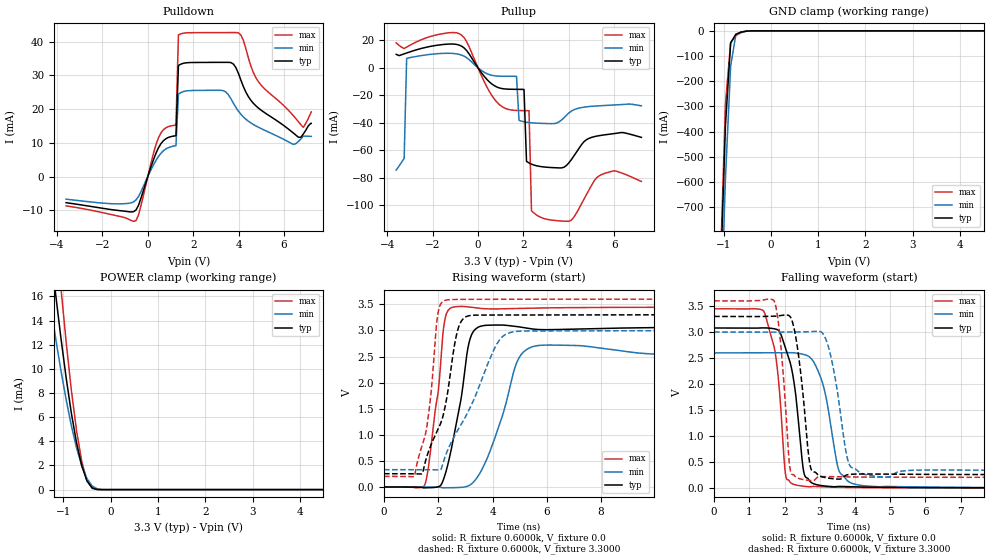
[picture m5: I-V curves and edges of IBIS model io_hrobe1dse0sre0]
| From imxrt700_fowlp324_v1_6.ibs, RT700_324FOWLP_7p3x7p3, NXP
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[Model] io_hrobe1dse0sre0
|   Model io_hrobe1dse0sre0
| This model was characterised for following simulation conditions:
| External (pad) voltage:
|   - Typ: 3.3V,   - Min: 3.0V,   - Max: 3.6V
| Library cells for typ/min/max conditions are connected as defined below:
|  PAD_IO - External Pad
|  ipp_do - Core Input
|  ipp_obe - Output Buffer Enable
|  ASRCN3V3[3] - NC
|  ASRCN3V3[4] - NC
|  ASRCP3V3[4] - NC
|  REFAPBIAS3V3 - gnde
|  REFBAMPL3V3 - vdd1v8
|  REFCAMPH3V3 - vdd1v8
|  REFDNBIAS3V3 - vdd1v8
|  REFH3V3 - REFH3V3
|  REFL3V3 - REFL3V3
|  gnde - gnde
|  ipp_dse - gnde
|  ipp_ina235_3v - NC
|  ipp_ina40_3v - NC
|  ipp_ina_mux - NC
|  ipp_ind - NC
|  ipp_ind_1p8v - NC
|  ipp_ind_3v - NC
|  ipp_sre - gnde
|  vdd - vdd
|  vdd1v8 - vdd1v8
|  vdda - vdde3v3
|  vdde3v3 - vdde3v3
| All other pins connected to ground
Model_type I/O
Polarity   Non-Inverting
Enable   Active-High
Vinl =   0.9900V
Vinh =   2.3100V
Vmeas =  1.6500V
Cref =   15.0000pF
Rref =   0.6000k
Vref =   0.0V
C_comp   4.0008pF   3.8189pF   4.1206pF
|C_comp_pullup   0.5645pF   0.7341pF   0.4703pF
|C_comp_pulldown   2.1156pF   2.2138pF   1.8992pF
[Model Spec]
| variable   typ   min   max
Vinh   2.3100V   NA   NA
Vinl   0.9900V   NA   NA
Vref   0.0V   0.0V   0.0V
Cref   15.0000pF   15.0000pF   15.0000pF
Rref   0.6000k   0.6000k   0.6000k
[Receiver Thresholds]
Vcross_high  =   0.0V
Vcross_low  =   0.0V
Vdiff_ac  =   0.0V
Vdiff_dc  =   0.0V
Tdiffslew_ac  =   0.0S
[Temperature Range]   25.0000   0.1250k   -40.0000
[Voltage Range]   3.3000V   3.0000V   3.6000V
[Pullup Reference]   3.3000V   3.0000V   3.6000V
[Pulldown Reference]   0.0V   0.0V   0.0V
[POWER Clamp Reference]   3.3000V   3.0000V   3.6000V
[GND Clamp Reference]   0.0V   0.0V   0.0V
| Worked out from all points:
|   slope of the pulldown table from 0 to 0.495 V, typ, clamps not added: 56.2 ohm
|   slope of the pullup table from 0 to 0.495 V, typ, clamps not added: 48.6 ohm
|   GND clamp passes 1 mA (typ) near -0.49 V on its own axis
|   POWER clamp passes 1 mA (typ) near -0.52 V on its own axis
|   rising waveform, R_fixture 0.6000k, V_fixture 0.0: 20-80 % time 596ps typ, 935ps min, 426ps max; typ from 0 V to 3.08 V
|   rising waveform, R_fixture 0.6000k, V_fixture 3.3000: 20-80 % time 811ps typ, 1.42ns min, 442ps max; typ from 0.254 V to 3.3 V
|   falling waveform, R_fixture 0.6000k, V_fixture 0.0: 20-80 % time 347ps typ, 425ps min, 283ps max; typ from 3.08 V to 0 V
|   falling waveform, R_fixture 0.6000k, V_fixture 3.3000: 20-80 % time 278ps typ, 365ps min, 222ps max; typ from 3.3 V to 0.254 V
[Pulldown]
|Voltage   I(typ)   I(min)   I(max)
-3.6V     -7.76mA    -6.72mA    -8.7mA
-520mV    -9.932mA   -6.949mA   -13.06mA
470mV     8.52mA     5.95mA     11.5mA
1.24V     12.09mA    9.145mA    15.23mA
1.35V     32.94mA    24.47mA    42.02mA
1.46V     33.35mA    24.92mA    42.34mA
3.33V     33.87mA    25.46mA    42.7mA
3.99V     30.63mA    19.41mA    42.61mA
5.09V     19.21mA    13.9mA     26.38mA
6.41V     12.92mA    9.507mA    18.07mA
6.85V     12.6mA     11.99mA    14.58mA
7.2V      15.78mA    11.9mA     19.19mA
[Pullup]
|Voltage   I(typ)   I(min)   I(max)
-3.6V     9.752mA    -74.51mA   18.1mA
-3.25V    10.1mA     -65.93mA   14.02mA
-3.14V    10.73mA    6.826mA    15.05mA
-830mV    16.51mA    9.731mA    24.85mA
1.7V      -15.72mA   -6.278mA   -31.08mA
1.81V     -15.74mA   -38.27mA   -31.14mA
2.03V     -15.78mA   -39.34mA   -31.22mA
2.14V     -68.17mA   -39.67mA   -31.25mA
2.25V     -69.31mA   -39.91mA   -31.27mA
2.36V     -70.19mA   -40.09mA   -104.1mA
2.69V     -71.74mA   -40.43mA   -108.3mA
7.2V      -50.7mA    -27.72mA   -82.8mA
[GND_clamp]
|Voltage   I(typ)   I(min)   I(max)
-3.6V     -19.67A    -19.55A    -20.65A
-1.07V    -1.013A    -1.224A    -956.3mA
-960mV    -377.1mA   -587.4mA   -291.7mA
-850mV    -48.21mA   -140.8mA   -46.94mA
-740mV    -13.57mA   -15.59mA   -19.22mA
-630mV    -5.137mA   -4.351mA   -7.235mA
-520mV    -1.276mA   -1.53mA    -1.554mA
-300mV    -4.403uA   -32.47uA   -997nA
7.2V      0A         0A         0A
[POWER_clamp]
|Voltage   I(typ)   I(min)   I(max)
-3.6V     102.5mA    81.21mA    131.1mA
-1.38V    23.81mA    18.18mA    31.78mA
-1.27V    19.88mA    15.26mA    26.56mA
-1.16V    16.12mA    12.48mA    21.52mA
-1.05V    12.56mA    9.868mA    16.71mA
-830mV    6.344mA    5.304mA    8.253mA
-720mV    3.878mA    3.458mA    4.888mA
-610mV    1.973mA    1.979mA    2.327mA
-500mV    725uA      918.2uA    733.4uA
-390mV    144.3uA    301.5uA    95.95uA
-170mV    198.2nA    4.056uA    20.28nA
7.2V      0A         0A         0A
[Ramp]
| variable   typ   min   max
dV/dt_r  1.8464/0.5956n   1.5590/0.9347n   2.0681/0.4255n
dV/dt_f  1.8274/0.2775n   1.6009/0.3654n   2.0384/0.2219n
R_load = 0.6000k
[Rising Waveform]
R_fixture= 0.6000k
V_fixture= 0.0
V_fixture_min= 0.0
V_fixture_max= 0.0
|time   V(typ)   V(min)   V(max)
0s        180nV      2.945uV    139nV
1.511ns   -16.45mV   -832.6uV   46.91mV
1.996ns   3.716mV    -4.935mV   1.812V
2.224ns   187.6mV    -16.17mV   3.147V
2.657ns   1.198V     -12.73mV   3.456V
3.104ns   2.689V     19.88mV    3.451V
3.341ns   3.009V     117.6mV    3.438V
4.935ns   3.072V     2.432V     3.422V
5.73ns    3.017V     2.713V     3.43V
60ns      3.077V     2.598V     3.447V
[Rising Waveform]
R_fixture= 0.6000k
V_fixture= 3.3000
V_fixture_min= 3.0000
V_fixture_max= 3.6000
|time   V(typ)   V(min)   V(max)
0s        254.3mV    331.8mV    202.7mV
1.129ns   253.9mV    331.7mV    211.9mV
1.608ns   628.1mV    331.7mV    1.251V
1.994ns   1.108V     327.7mV    3.338V
2.384ns   1.94V      751mV      3.589V
2.675ns   2.918V     1.047V     3.594V
2.917ns   3.223V     1.261V     3.595V
4.139ns   3.295V     2.721V     3.596V
4.896ns   3.295V     2.982V     3.598V
60ns      3.3V       3V         3.6V
[Falling Waveform]
R_fixture= 0.6000k
V_fixture= 0.0
V_fixture_min= 0.0
V_fixture_max= 0.0
|time   V(typ)   V(min)   V(max)
0s        3.077V     2.599V     3.447V
1.406ns   3.08V      2.599V     3.403V
1.861ns   3.003V     2.598V     1.829V
2.049ns   2.647V     2.603V     191.1mV
2.534ns   350.7mV    2.571V     31.8mV
2.672ns   173.3mV    2.536V     21.7mV
3.123ns   37.11mV    1.911V     18.6mV
3.557ns   27.27mV    311.7mV    10.01mV
4.49ns    12.42mV    28.03mV    3.324mV
60ns      676.4nV    2.172uV    497.9nV
[Falling Waveform]
R_fixture= 0.6000k
V_fixture= 3.3000
V_fixture_min= 3.0000
V_fixture_max= 3.6000
|time   V(typ)   V(min)   V(max)
0s        3.3V       3V         3.6V
1.715ns   3.303V     3V         3.583V
1.886ns   3.317V     2.998V     2.804V
2.164ns   3.292V     3.001V     335.7mV
2.388ns   2.6V       3.001V     184.2mV
2.761ns   349.9mV    3.009V     138.8mV
3.254ns   185.8mV    2.693V     216.1mV
3.854ns   259.3mV    428.5mV    209.9mV
4.778ns   264.6mV    210.4mV    205.5mV
60ns      254.3mV    331.8mV    202.7mV
